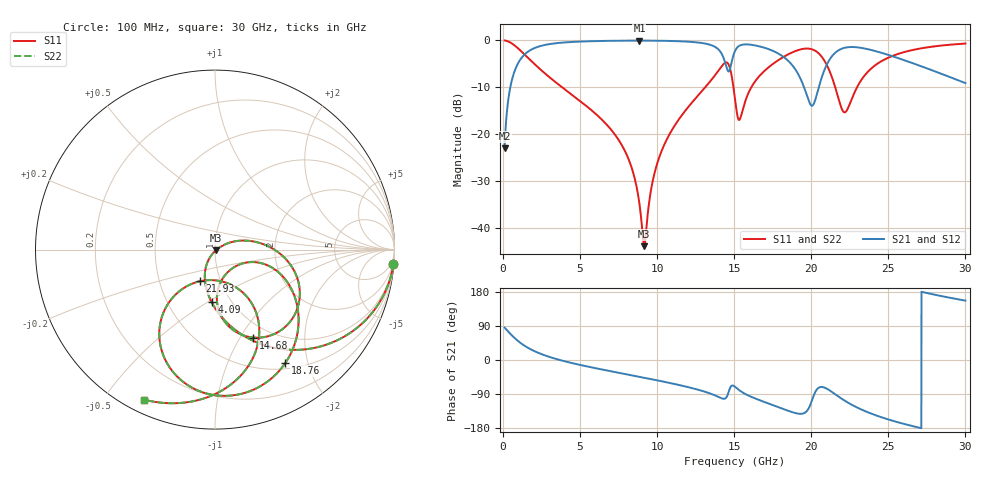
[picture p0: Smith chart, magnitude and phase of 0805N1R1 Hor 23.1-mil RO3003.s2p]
# GHz S MA R 50
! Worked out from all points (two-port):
!   3201 points, 100 MHz to 30 GHz, reference 50 ohm
!   highest |S21| = -0.06 dB at 8.846 GHz (marker M1); lowest = -23.0 dB at 100 MHz (marker M2)
!   |S21| within 3 dB of the highest: 1.384 GHz to 14.22 GHz (12.83 GHz wide, 165 % of centre); 21.43 GHz to 24.95 GHz (3.527 GHz wide, 15.2 % of centre)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
!   lowest |S11| = -43.9 dB at 9.163 GHz (marker M3), VSWR 1.01, Z = 50.4 - j0.472 ohm
!   |S11| at or under -10 dB: 3.828 GHz to 13.12 GHz (9.29 GHz wide, 110 % of centre); 14.95 GHz to 16.11 GHz (1.161 GHz wide, 7.48 % of centre); 21.55 GHz to 22.97 GHz (1.416 GHz wide, 6.36 % of centre)
!   |S22| runs from -43.9 to 0.0 dB; largest |S21 - S12| = 0
!   S11 on the Smith chart (normalised r, x): 100 MHz: 1, -25; 4.09 GHz: 0.81, -0.52; 14.68 GHz: 0.83, -1.14; 18.76 GHz: 0.58, -1.64; 21.93 GHz: 0.80, -0.29; 30 GHz: 0.06, -0.63
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0.1  0.9975 -4.6  0.07072 85.4  0.07072 85.4  0.9975 -4.6
0.4830937  0.9458 -21.5  0.3243 68.5  0.3243 68.5  0.9458 -21.5
1.090437  0.7888 -43.6  0.6136 46.3  0.6136 46.3  0.7888 -43.6
4.089781  0.2931 -93.7  0.9528 -4.3  0.9528 -4.3  0.2931 -93.7
5.089563  0.2195 -102.9  0.9717 -13.8  0.9717 -13.8  0.2195 -102.9
7.715156  0.07579 -121.5  0.9917 -35.4  0.9917 -35.4  0.07579 -121.5
8.84575  0.01824 -114.8  0.9934 -44.3  0.9934 -44.3  0.01824 -114.8
9.163438  0.006388 -47.0  0.9933 -46.9  0.9933 -46.9  0.006388 -47.0
10.06978  0.05275 27.6  0.9908 -54.2  0.9908 -54.2  0.05275 27.6
13.27469  0.3389 -0.9  0.912 -86.1  0.912 -86.1  0.3389 -0.9
14.24644  0.5439 -29.9  0.6871 -101.9  0.6871 -101.9  0.5439 -29.9
14.67625  0.5334 -66.7  0.4724 -79.5  0.4724 -79.5  0.5334 -66.7
15.05  0.2371 -86.7  0.7696 -70.6  0.7696 -70.6  0.2371 -86.7
15.35834  0.1435 -44.4  0.8801 -80.6  0.8801 -80.6  0.1435 -44.4
16.20863  0.3366 -17.7  0.8915 -99.0  0.8915 -99.0  0.3366 -17.7
18.75947  0.7435 -58.2  0.5446 -137.6  0.5446 -137.6  0.7435 -58.2
20.03956  0.8034 -93.2  0.2006 -107.1  0.2006 -107.1  0.8034 -93.2
20.93656  0.5745 -122.7  0.5208 -74.3  0.5208 -74.3  0.5745 -122.7
21.927  0.1963 -115.7  0.8083 -101.0  0.8083 -101.0  0.1963 -115.7
23.30988  0.3914 -56.1  0.8276 -131.8  0.8276 -131.8  0.3914 -56.1
25.01978  0.6561 -72.2  0.6977 -157.2  0.6977 -157.2  0.6561 -72.2
30  0.9243 -115.2  0.3502 156.7  0.3502 156.7  0.9243 -115.2
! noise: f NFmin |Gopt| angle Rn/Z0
0.1  0.001376  0.9585  1.332  0.007476
3.417  0.007656  0.7497  18.81  0.006001
6.743  0.0133  0.7237  35.26  0.008701
10.06  0.02038  0.7351  51.05  0.01258
13.39  0.0505  0.8519  66.54  0.05098
16.7  0.0687  0.8662  81.41  0.06363
20.03  0.6244  0.9816  95.95  3.475
23.35  0.1161  0.8912  109.4  0.07804
26.67  0.1007  0.8615  121.9  0.0374
30  0.1152  0.8671  134.1  0.02916
